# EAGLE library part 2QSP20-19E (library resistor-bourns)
BOURNS RESISTOR NETWORK
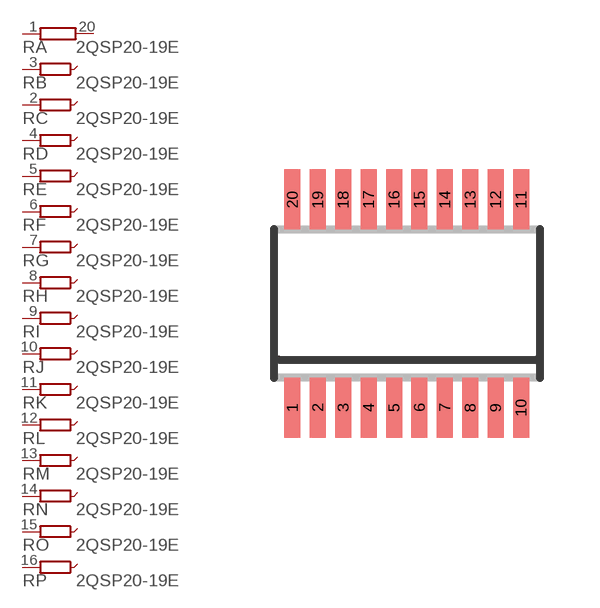
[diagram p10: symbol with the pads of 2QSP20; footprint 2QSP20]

Designator prefix R; gates A=R1NV B=R1NVXX C=R1NVXX D=R1NVXX E=R1NVXX F=R1NVXX G=R1NVXX H=R1NVXX I=R1NVXX J=R1NVXX K=R1NVXX L=R1NVXX M=R1NVXX N=R1NVXX O=R1NVXX P=R1NVXX Q=R1NVXX R=R1NVXX S=R1NVXX

## 2QSP20-19E (OC_FARNELL: unknown; OC_NEWARK: unknown)  [2QSP20]
1  A:1  pas
2  C:1  pas
3  B:1  pas
4  D:1  pas
5  E:1  pas
6  F:1  pas
7  G:1  pas
8  H:1  pas
9  I:1  pas
10  J:1  pas
11  K:1  pas
12  L:1  pas
13  M:1  pas
14  N:1  pas
15  O:1  pas
16  P:1  pas
17  Q:1  pas
18  R:1  pas
19  S:1  pas
20  A:2  pas

## Footprint 2QSP20 (pad centres in mm)
BOURNS RESISTOR NETWORK
smd 0.4 x 1.5: 1 -2.223,-2.6; 2 -1.588,-2.6; 3 -0.953,-2.6; 4 -0.318,-2.6; 5 0.318,-2.6; 6 0.953,-2.6; 7 1.588,-2.6; 8 2.223,-2.6; 9 2.858,-2.6; 10 3.493,-2.6; 11 3.493,2.6; 12 2.858,2.6; 13 2.223,2.6; 14 1.588,2.6; 15 0.953,2.6; 16 0.318,2.6; 17 -0.318,2.6; 18 -0.953,2.6; 19 -1.588,2.6; 20 -2.223,2.6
